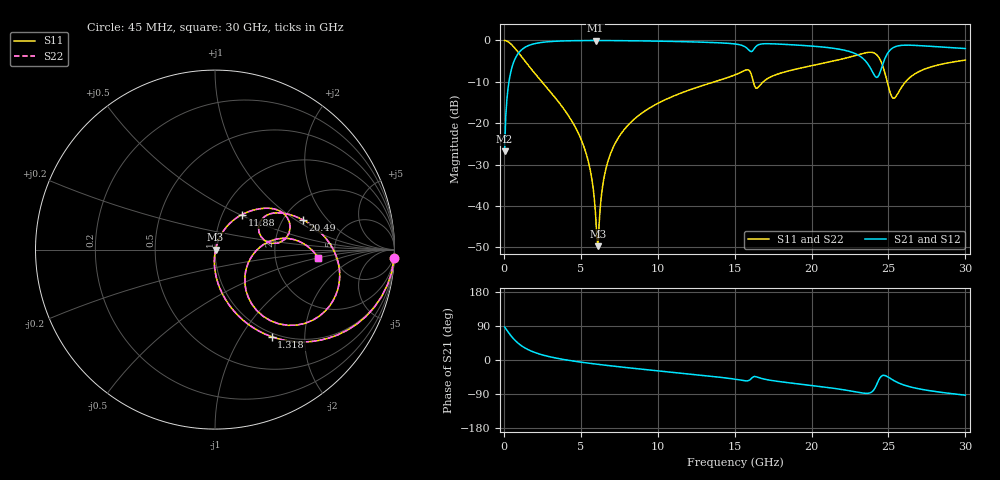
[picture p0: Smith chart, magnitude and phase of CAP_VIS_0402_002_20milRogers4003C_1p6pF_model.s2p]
! S-parameter model data by Modelithics Inc.  support@modelithics.com  813-866-6335  Tampa FL USA
! S-Parameter data specifications:
! Substrate: 20-mil Rogers 4003C, substrate thickness, H=0.508mm, Dielectric constant, Er=3.75
! PCB Mounting Pad Footprint: Pad width, PadW=0.50mm , Pad length, PadL=0.50mm , Pad gap, PadG (edge-to-edge)=0.40mm , Reference planes=1.4mm apart
! Created Wed Nov 18 12:42:44 2015
# hz S ma R 50
! 2 Port Network Data from SP1.SP block
! freq  magS11  angS11  magS21  angS21  magS12  angS12  magS22  angS22
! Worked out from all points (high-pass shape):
!   401 points, 45 MHz to 30 GHz, reference 50 ohm
!   highest |S21| = -0.03 dB at 5.961 GHz (marker M1); lowest = -26.8 dB at 45 MHz (marker M2)
!   |S21| within 3 dB of the highest: 957 MHz to 22.73 GHz (21.78 GHz wide, 184 % of centre); 24.96 GHz to end of sweep
!   lowest |S11| = -49.7 dB at 6.111 GHz (marker M3), VSWR 1.01, Z = 50.3 + j0.0339 ohm
!   |S11| at or under -10 dB: 2.468 GHz to 13.69 GHz (11.22 GHz wide, 139 % of centre); 16.21 GHz to 16.86 GHz (643.6 MHz wide, 3.89 % of centre); 24.92 GHz to 26.11 GHz (1.194 GHz wide, 4.68 % of centre)
!   |S22| runs from -49.7 to 0.0 dB; largest |S21 - S12| = 0
!   S11 on the Smith chart (normalised r, x): 45 MHz: 1, -42; 1.318 GHz: 0.94, -1.38; 11.88 GHz: 1.23, +0.51; 20.49 GHz: 2.54, +1.15; 30 GHz: 3.67, -0.51
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4.5e7  0.999 -2.7  0.04575 87.3  0.04575 87.3  0.999 -2.7
4.94325e8  0.892 -27.8  0.4516 62.2  0.4516 62.2  0.892 -27.8
1.318088e9  0.5791 -57.0  0.814 32.9  0.814 32.9  0.5791 -57.0
2.591175e9  0.2972 -77.2  0.9528 12.5  0.9528 12.5  0.2972 -77.2
5.062462e9  0.06077 -93.3  0.9952 -6.0  0.9952 -6.0  0.06077 -93.3
5.661562e9  0.02424 -92.1  0.9965 -9.2  0.9965 -9.2  0.02424 -92.1
5.961112e9  0.007801 -77.5  0.9967 -10.7  0.9967 -10.7  0.007801 -77.5
6.110888e9  0.003265 5.9  0.9967 -11.4  0.9967 -11.4  0.003265 5.9
6.560212e9  0.02459 68.8  0.9963 -13.6  0.9963 -13.6  0.02459 68.8
7.159312e9  0.05367 70.0  0.9949 -16.4  0.9949 -16.4  0.05367 70.0
1.007992e10  0.1765 59.7  0.9797 -28.9  0.9797 -28.9  0.1765 59.7
1.187722e10  0.2449 52.5  0.9641 -36.3  0.9641 -36.3  0.2449 52.5
1.50225e10  0.3835 36.9  0.9059 -50.6  0.9059 -50.6  0.3835 36.9
1.584626e10  0.442 20.4  0.7911 -54.9  0.7911 -54.9  0.442 20.4
1.644536e10  0.2639 21.8  0.8645 -44.7  0.8645 -44.7  0.2639 21.8
2.003996e10  0.4965 21.1  0.8537 -67.4  0.8537 -67.4  0.4965 21.1
2.048929e10  0.517 18.7  0.84 -69.6  0.84 -69.6  0.517 18.7
2.370945e10  0.7176 -16.2  0.504 -87.7  0.504 -87.7  0.7176 -16.2
2.445832e10  0.5853 -46.1  0.4139 -46.4  0.4139 -46.4  0.5853 -46.1
2.505742e10  0.2517 -48.6  0.7475 -47.0  0.7475 -47.0  0.2517 -48.6
2.633051e10  0.3482 9.7  0.8762 -70.0  0.8762 -70.0  0.3482 9.7
3e10  0.5782 -4.6  0.7976 -92.9  0.7976 -92.9  0.5782 -4.6
